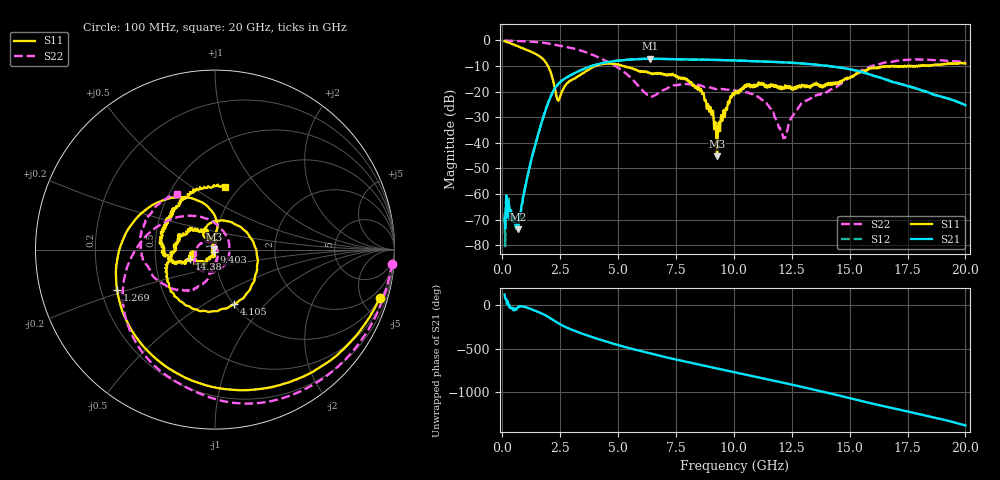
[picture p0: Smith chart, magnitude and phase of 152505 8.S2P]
!  2-Port S-parameters saved by WinCal
! VAR MeasName=S-Parameters (CALIBRATED_DATA) read from VNA (N5230C)
! VAR MeasDate=4/10/2015 9:29:09 AM
! VAR NAME=152505 8
! VAR FILENAME=152505 8.S2P
! VAR DATE=4/10/2015 9:29:09 AM
! VAR PHYS_PORTS=1,2
# Hz S DB R 50
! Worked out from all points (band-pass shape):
!   801 points, 100 MHz to 20 GHz, reference 50 ohm
!   highest |S21| = -7.23 dB at 6.393 GHz (marker M1); lowest = -73.8 dB at 672.1 MHz (marker M2)
!   |S21| within 3 dB of the highest: 3.794 GHz to 14.25 GHz (10.46 GHz wide, 116 % of centre)
!   lowest |S11| = -45.2 dB at 9.279 GHz (marker M3), VSWR 1.01, Z = 49.5 + j0.262 ohm
!   |S11| at or under -10 dB: 1.972 GHz to 4.049 GHz (2.077 GHz wide, 69 % of centre); 5.214 GHz to 16.86 GHz (11.64 GHz wide, 106 % of centre); 16.87 GHz to 17.37 GHz (503.9 MHz wide, 2.94 % of centre)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
!   |S22| runs from -38.2 to -0.1 dB; largest |S21 - S12| = 0.0056
!   S11 on the Smith chart (normalised r, x): 100 MHz: 1.06, -6.80; 1.269 GHz: 0.27, -0.19; 4.105 GHz: 1.01, -0.69; 9.403 GHz: 0.99, -0.03; 14.38 GHz: 0.75, -0.08; 20 GHz: 0.87, +0.69
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1e8  -0.38 -16.3  -69.49 122.9  -67.60 121.4  -0.09 -4.6
2.74125e8  -0.92 -41.0  -63.20 -3.4  -61.76 -7.5  -0.17 -11.5
6.72125e8  -2.33 -91.3  -73.79 -32.2  -72.33 -25.7  -0.32 -27.3
1.269125e9  -4.57 -157.4  -46.02 -48.0  -46.00 -47.9  -0.59 -51.4
1.84125e9  -8.21 133.5  -28.04 -113.7  -28.04 -113.8  -1.07 -75.6
2.413375e9  -23.57 112.0  -17.08 153.0  -17.10 153.1  -2.02 -99.5
3.43325e9  -13.17 7.2  -11.53 32.9  -11.51 33.2  -4.12 -143.6
4.104875e9  -9.80 -70.5  -9.39 -28.0  -9.36 -27.8  -6.48 -173.6
5.099875e9  -9.62 -141.5  -7.88 -107.8  -7.88 -108.1  -11.31 137.7
6.393375e9  -12.94 -178.3  -7.23 162.1  -7.24 161.9  -21.87 6.3
6.741625e9  -12.74 174.0  -7.28 139.5  -7.24 139.1  -20.65 -44.9
7.61225e9  -14.96 150.8  -7.39 85.7  -7.46 85.8  -17.51 -112.0
8.582375e9  -19.02 114.7  -7.59 29.5  -7.56 29.3  -17.72 -151.7
9.278875e9  -45.23 151.1  -7.68 -10.7  -7.69 -10.7  -19.03 -164.6
9.40325e9  -35.49 -113.2  -7.69 -18.0  -7.72 -17.9  -18.99 -165.4
1.005e10  -20.05 -128.7  -7.88 -55.5  -7.87 -55.5  -19.56 -178.2
1.141812e10  -17.97 -162.7  -8.38 -133.5  -8.37 -133.7  -24.61 130.0
1.216438e10  -18.92 -172.7  -8.64 -176.8  -8.60 -177.0  -38.05 26.9
1.338325e10  -17.73 -167.1  -9.41 109.6  -9.37 109.7  -22.11 -93.5
1.437825e10  -16.40 -159.8  -10.41 47.9  -10.37 47.5  -18.40 -99.4
1.669162e10  -10.32 167.2  -15.70 -98.9  -15.78 -99.9  -8.48 -158.1
2e10  -9.08 80.8  -25.36 51.8  -25.37 52.1  -8.49 124.3
